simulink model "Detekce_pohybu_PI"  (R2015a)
settings: Solver=ode45  StartTime=0.0  StopTime=10.0  RelTol=1e-3
undefined symbols (not defined in the file or in its folder): Rec, SDTV
libraries: embdlinuxlib x2, visionconversions x1

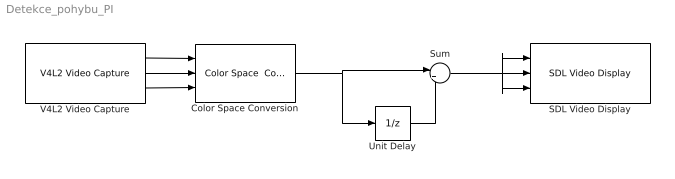
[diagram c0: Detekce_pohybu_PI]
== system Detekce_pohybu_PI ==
  Color Space Conversion : visionconversions/Color Space  Conversion  conversion=Obsolete  conversionActive=R'G'B' to intensity  wp_str=D65  rec=Rec. 601 (SDTV)  sys=1125/60/2:1  imagePorts=Separate color signals
  SDL Video Display : embdlinuxlib/SDL Video Display  pixelFormat=RGB  pixelOrder=Planar  rowMajor=on  blockPlatform=Raspberry Pi
  Sum : Sum  Inputs=|+-
  Unit Delay : UnitDelay  SampleTime=-1
  V4L2 Video Capture : embdlinuxlib/V4L2 Video Capture  m_devName='/dev/video0'  roi=[0, 0, 640, 480]  imSizeSelection=640x480  imSize=[640, 480]  pixelFormat=RGB  pixelOrder=Planar  sampleTime=1/10  simOutput=Colorbars  blockPlatform=Raspberry Pi
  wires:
  V4L2 Video Capture/3 -> Color Space Conversion/3
  V4L2 Video Capture/2 -> Color Space Conversion/2
  V4L2 Video Capture/1 -> Color Space Conversion/1
  Color Space Conversion/1 -> Sum/1, Unit Delay/1
  Sum/1 -> SDL Video Display/3, SDL Video Display/1, SDL Video Display/2
  Unit Delay/1 -> Sum/2
